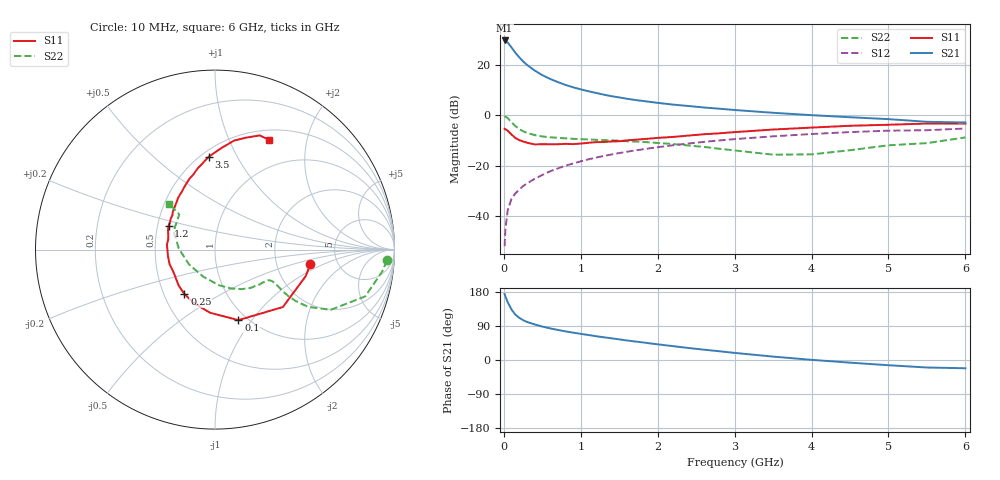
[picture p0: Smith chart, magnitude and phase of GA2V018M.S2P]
! Infineon Technologies  Discrete & RF Semiconductors
! BF775
! Si NPN RF Bipolar Junction Transistor in SOT23
! VCE = 2 V  IC = 18 mA
! Common Emitter S-Parameters:  May  1996
# GHz  S  MA  R  50
!  f  S11  S21  S12  S22
! GHz  MAG  ANG  MAG  ANG  MAG  ANG  MAG  ANG
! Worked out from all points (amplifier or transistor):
!   36 points, 10 MHz to 6 GHz, reference 50 ohm
!   highest |S21| = 29.7 dB at 10 MHz (marker M1)
!   |S21| within 3 dB of that: start of sweep to 105.2 MHz
!   unconditionally stable (mu >= 1): 363.8 MHz to 3.833 GHz
!   at 250 MHz: K = 0.87, MSG = 24.8 dB, |S12| = -28.2 dB
!   at 1.4 GHz: K = 1.14, MAG = 9.3 dB, |S12| = -15.6 dB
!   at 6 GHz: K = 0.99, MSG = 1.2 dB, |S12| = -5.3 dB
!   S11 on the Smith chart (normalised r, x): 10 MHz: 3.15, -0.71; 100 MHz: 0.91, -0.86; 250 MHz: 0.64, -0.35; 1.2 GHz: 0.57, +0.17; 3.5 GHz: 0.55, +0.78; 6 GHz: 0.62, +1.42
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0.01  0.5379 -8.6  30.59 174.0  0.0025 84.8  0.9601 -3.6
0.02  0.5263 -16.4  30.22 168.1  0.0053 85.4  0.9401 -7.4
0.05  0.4955 -40.2  27.88 152.6  0.0129 74.3  0.8767 -17.3
0.1  0.4141 -71.6  22.21 133.1  0.022 66.7  0.7267 -27.5
0.15  0.3529 -94.5  17.46 119.6  0.028 64.4  0.6088 -31.6
0.2  0.3205 -111.6  14.17 111.4  0.0333 64.3  0.5313 -32.5
0.25  0.3004 -124.6  11.76 105.2  0.039 64.6  0.4801 -32.3
0.3  0.2844 -135.5  10.04 100.5  0.0442 65.9  0.4456 -31.6
0.4  0.2634 -151.0  7.751 93.9  0.0544 67.3  0.4034 -30.1
0.5  0.2658 -162.0  6.257 88.2  0.065 68.4  0.3787 -29.1
0.6  0.2645 -172.2  5.282 83.5  0.0767 68.5  0.3648 -28.9
0.7  0.265 -179.9  4.565 79.4  0.0875 68.9  0.3553 -29.1
0.8  0.2696 174.2  4.008 75.6  0.0989 68.0  0.3471 -29.5
0.9  0.2667 167.8  3.592 72.2  0.1102 67.6  0.3396 -30.3
1.1  0.2834 157.5  2.994 66.0  0.133 66.3  0.3302 -32.9
1.2  0.2916 152.6  2.769 62.8  0.144 65.3  0.3244 -34.2
1.6  0.3166 137.9  2.124 51.6  0.1879 61.0  0.3044 -41.3
2.2  0.3702 120.3  1.625 36.5  0.2529 53.9  0.2676 -55.3
3.5  0.5196 93.7  1.118 9.0  0.3807 36.2  0.1646 -113.3
4.5  0.617 80.0  0.912 -7.0  0.462 22.3  0.2016 178.4
5.5  0.6834 68.6  0.74 -19.8  0.5035 7.8  0.279 135.5
6  0.6818 63.6  0.717 -21.8  0.5443 3.6  0.3621 135.0
